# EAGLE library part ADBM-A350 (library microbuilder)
ADBM-A350 - Optical Finger Navigation Sensor VDD: 1.7-2.1V (1.8V Typical) VDDIO: 1.65-3.6V (1.8V or 2.8V Typical) Operating Temp: -20-70°C FPC Connector: Hirose FH26-17S-0.3SHW(05)
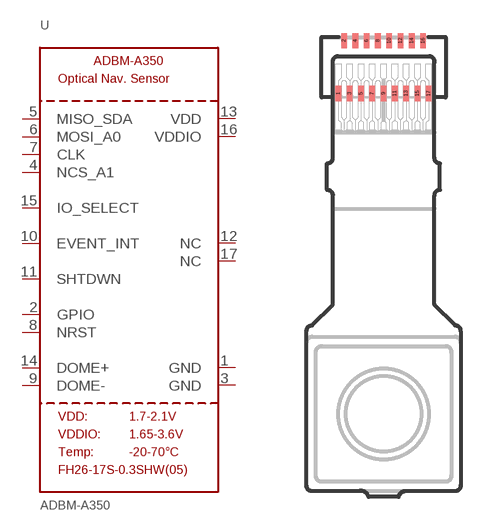
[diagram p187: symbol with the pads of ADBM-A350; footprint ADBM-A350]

Designator prefix U

## ADBM-A350  [ADBM-A350]
1  GND  pwr
2  GPIO  in
3  GND  pwr
4  NCS_A1  in
5  MISO_SDA  in
6  MOSI_A0  in
7  CLK  in
8  NRST  in
9  DOME-  in
10  EVENT_INT  in
11  SHTDWN  in
12  NC  nc
13  VDD  pwr
14  DOME+  in
15  IO_SELECT  in
16  VDDIO  pwr
17  NC  nc

## Footprint ADBM-A350 (pad centres in mm)
ADBM-A350 - Outline Only
smd 0.3 x 0.8: 1 -2.4,16.38; 2 -2.1,19.18; 3 -1.8,16.38; 4 -1.5,19.18; 5 -1.2,16.38; 6 -0.9,19.18; 7 -0.6,16.38; 8 -0.3,19.18; 9 0,16.38; 10 0.3,19.18; 11 0.6,16.38; 12 0.9,19.18; 13 1.2,16.38; 14 1.5,19.18; 15 1.8,16.38; 16 2.1,19.18; 17 2.4,16.38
